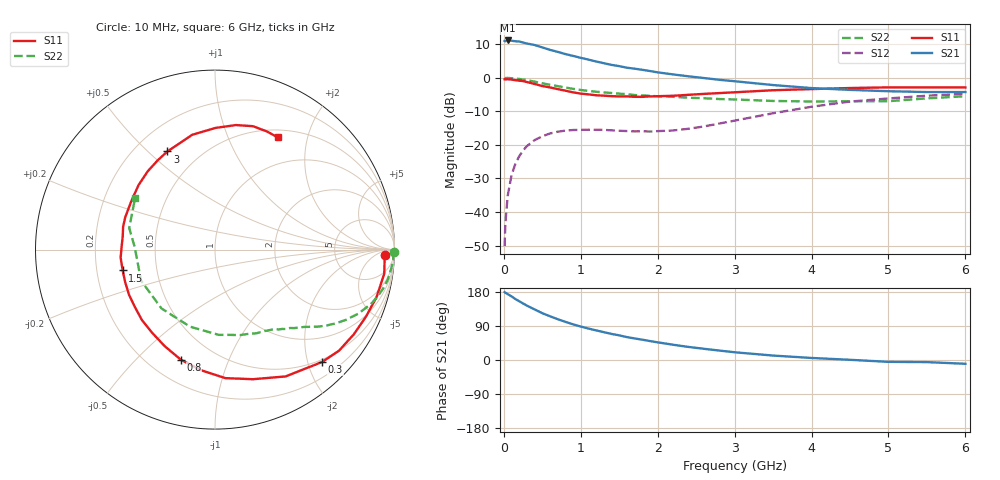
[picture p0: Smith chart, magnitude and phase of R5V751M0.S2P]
! SIEMENS Small Signal Semiconductors
! BFR183
! Si NPN RF Bipolar Junction Transistor in SOT23
! VCE = 0.75 V  IC = 1 mA
! Common Emitter S-Parameters:  May  1996
# GHz  S  MA  R  50
!  f  S11  S21  S12  S22
! GHz  MAG  ANG  MAG  ANG  MAG  ANG  MAG  ANG
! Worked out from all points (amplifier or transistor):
!   36 points, 10 MHz to 6 GHz, reference 50 ohm
!   highest |S21| = 11.1 dB at 50 MHz (marker M1)
!   |S21| within 3 dB of that: start of sweep to 632.9 MHz
!   unconditionally stable (mu >= 1): 1.612 GHz to 3.338 GHz
!   at 250 MHz: K = 0.16, MSG = 16.1 dB, |S12| = -21.7 dB
!   at 1.4 GHz: K = 0.88, MSG = 9.8 dB, |S12| = -15.7 dB
!   at 6 GHz: K = 1.00, MSG = 0.3 dB, |S12| = -4.8 dB
!   S11 on the Smith chart (normalised r, x): 10 MHz: 29, -17; 300 MHz: 0.45, -2.26; 800 MHz: 0.33, -0.68; 1.5 GHz: 0.31, -0.10; 3 GHz: 0.33, +0.58; 6 GHz: 0.60, +1.54
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0.01  0.9502 -1.7  3.534 179.1  0.0031 88.9  0.9964 -0.7
0.02  0.9465 -3.1  3.495 177.5  0.0068 88.5  0.9914 -1.3
0.05  0.9525 -8.1  3.596 173.8  0.0174 85.0  0.9953 -3.4
0.1  0.9384 -16.2  3.564 167.9  0.0353 80.3  0.9855 -6.8
0.15  0.9206 -23.9  3.498 160.9  0.0523 75.4  0.9764 -10.1
0.2  0.9061 -31.4  3.469 155.0  0.0679 70.6  0.9602 -13.3
0.3  0.8649 -46.4  3.233 143.4  0.0959 62.5  0.9221 -19.0
0.4  0.8087 -60.9  3.078 133.5  0.1179 54.8  0.8756 -24.0
0.5  0.7524 -73.7  2.831 123.5  0.1344 48.1  0.8268 -28.3
0.6  0.7184 -85.4  2.604 115.4  0.1479 42.7  0.7871 -31.5
0.8  0.6425 -107.2  2.254 100.7  0.1632 34.0  0.7166 -36.8
0.9  0.6066 -117.5  2.117 94.1  0.1666 31.3  0.6834 -39.0
1.1  0.5654 -136.1  1.865 83.0  0.1681 26.8  0.6377 -42.9
1.5  0.5275 -167.3  1.49 65.0  0.1622 23.6  0.5796 -49.7
1.8  0.5195 171.6  1.314 53.6  0.1599 27.0  0.5463 -54.7
2.2  0.5387 150.0  1.122 40.3  0.1639 34.4  0.5206 -63.5
3  0.6076 115.9  0.888 20.4  0.2298 46.1  0.4755 -87.5
3.5  0.6522 101.2  0.779 11.7  0.2964 44.7  0.4514 -108.0
4.5  0.7035 80.5  0.66 0.5  0.442 31.6  0.4467 -157.2
5  0.7194 72.9  0.63 -4.9  0.4924 21.9  0.4479 178.1
5.5  0.7189 66.4  0.613 -5.6  0.5406 16.0  0.4932 165.8
6  0.7166 60.8  0.613 -10.0  0.5766 6.5  0.5308 146.9
